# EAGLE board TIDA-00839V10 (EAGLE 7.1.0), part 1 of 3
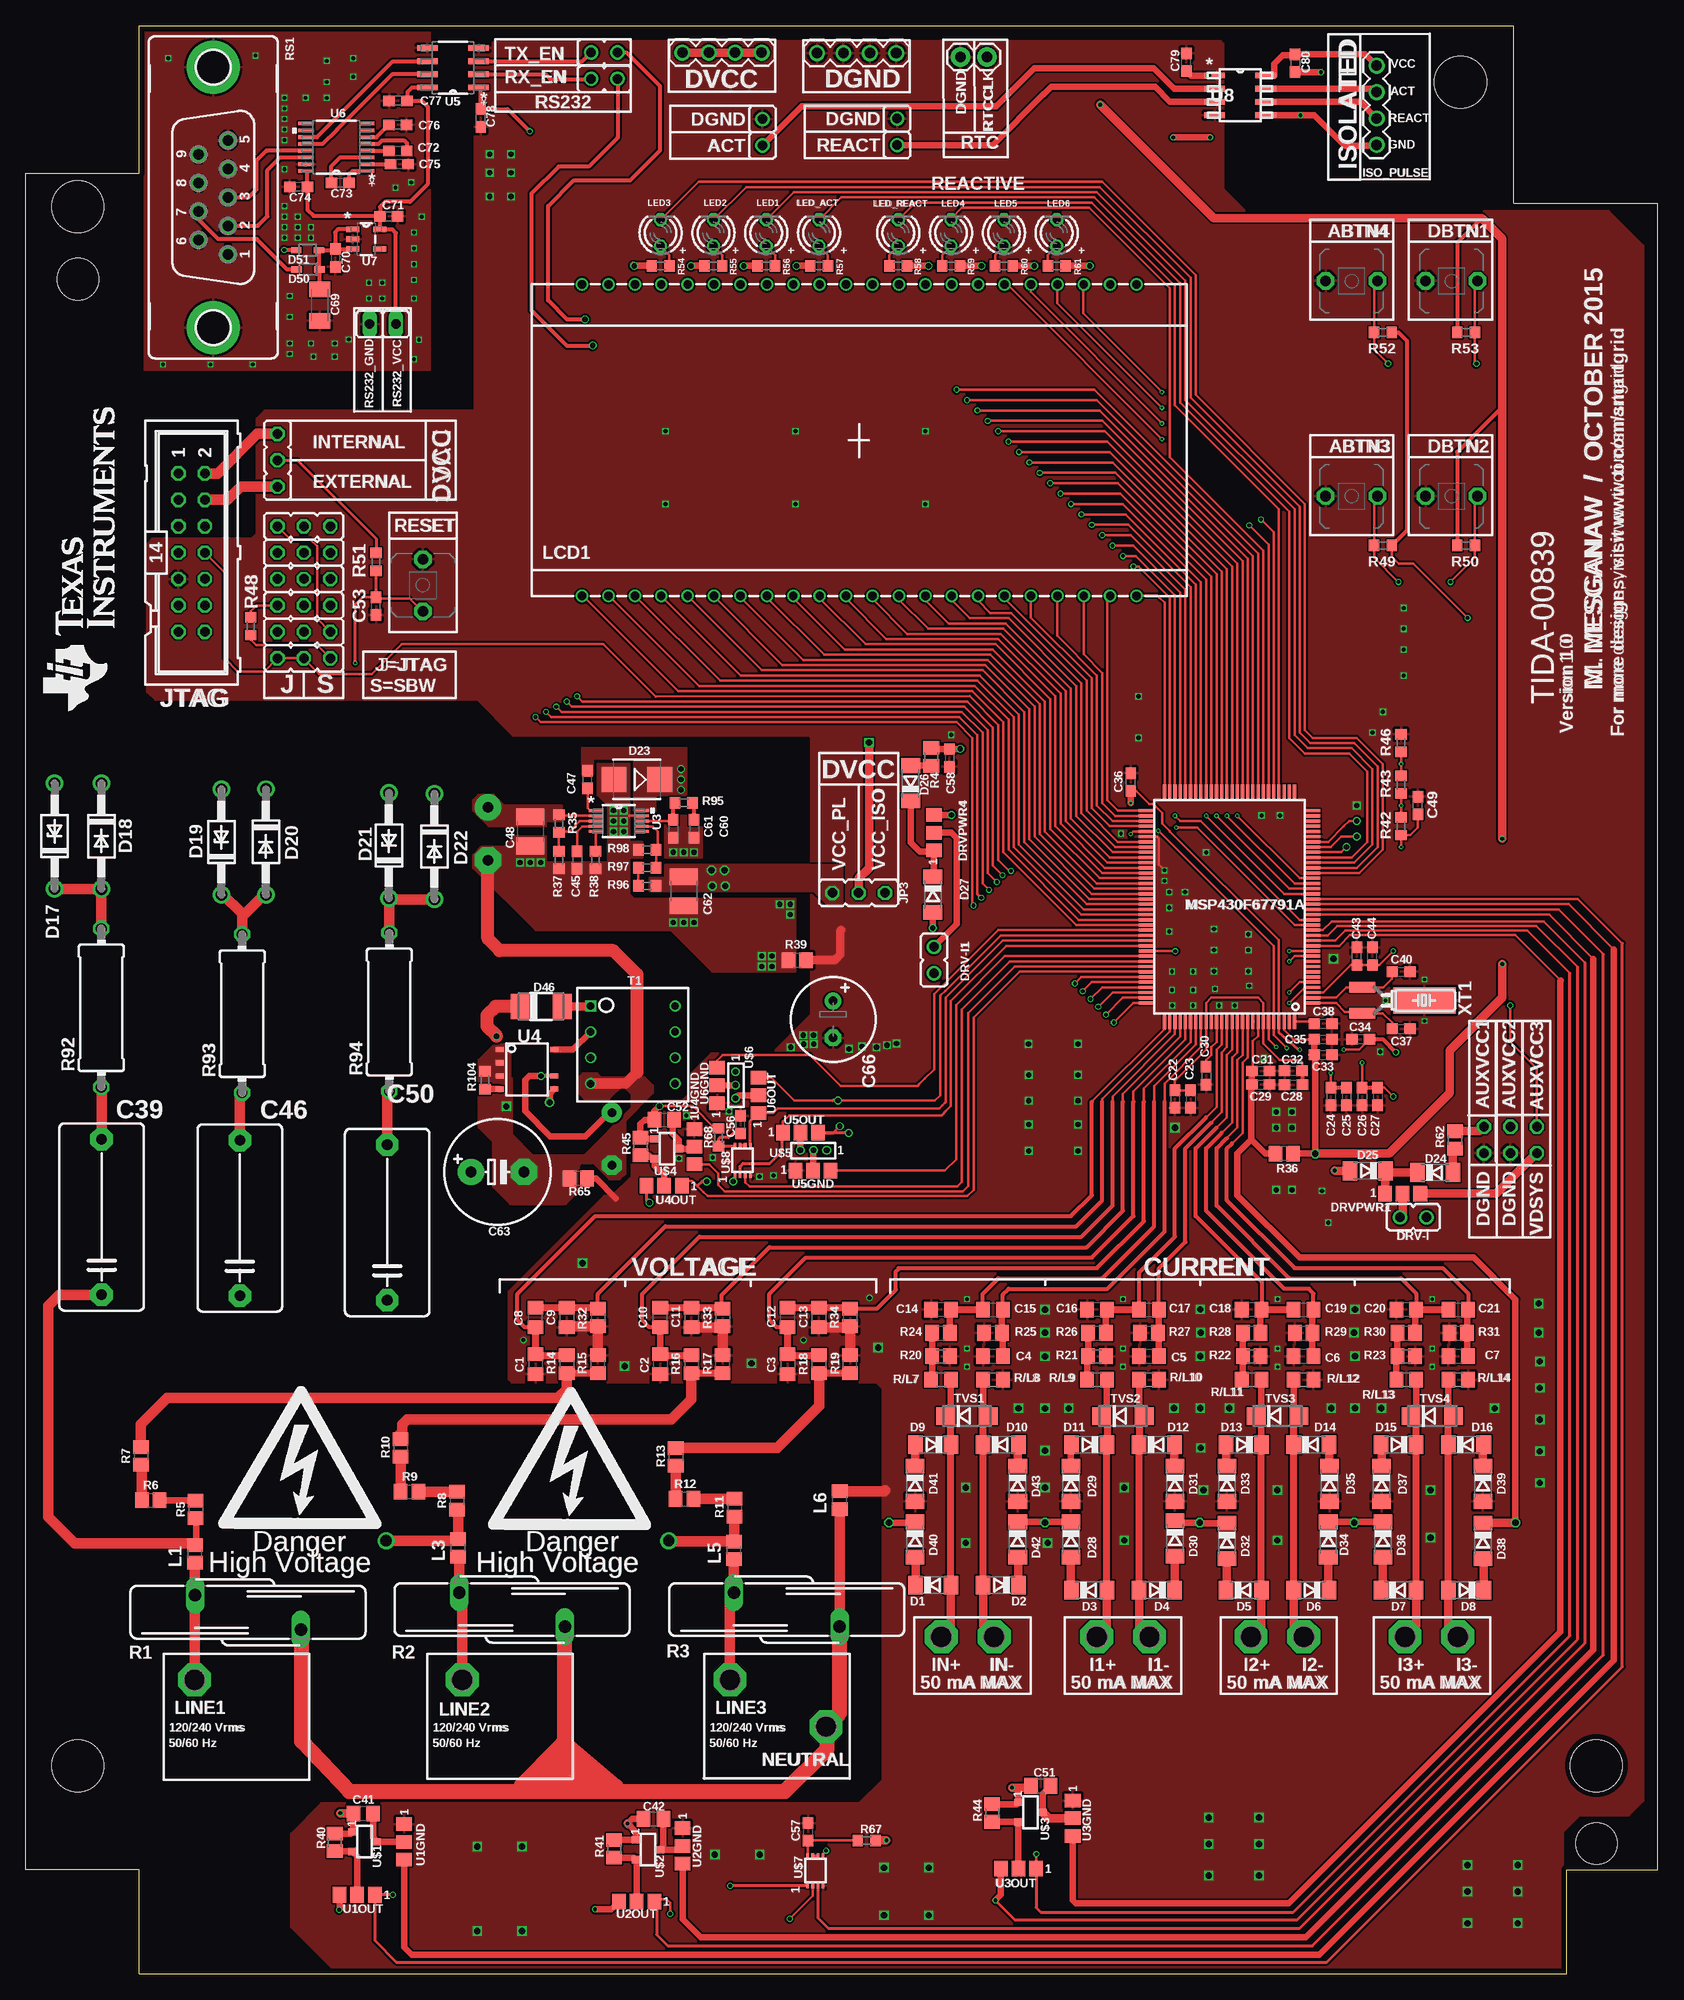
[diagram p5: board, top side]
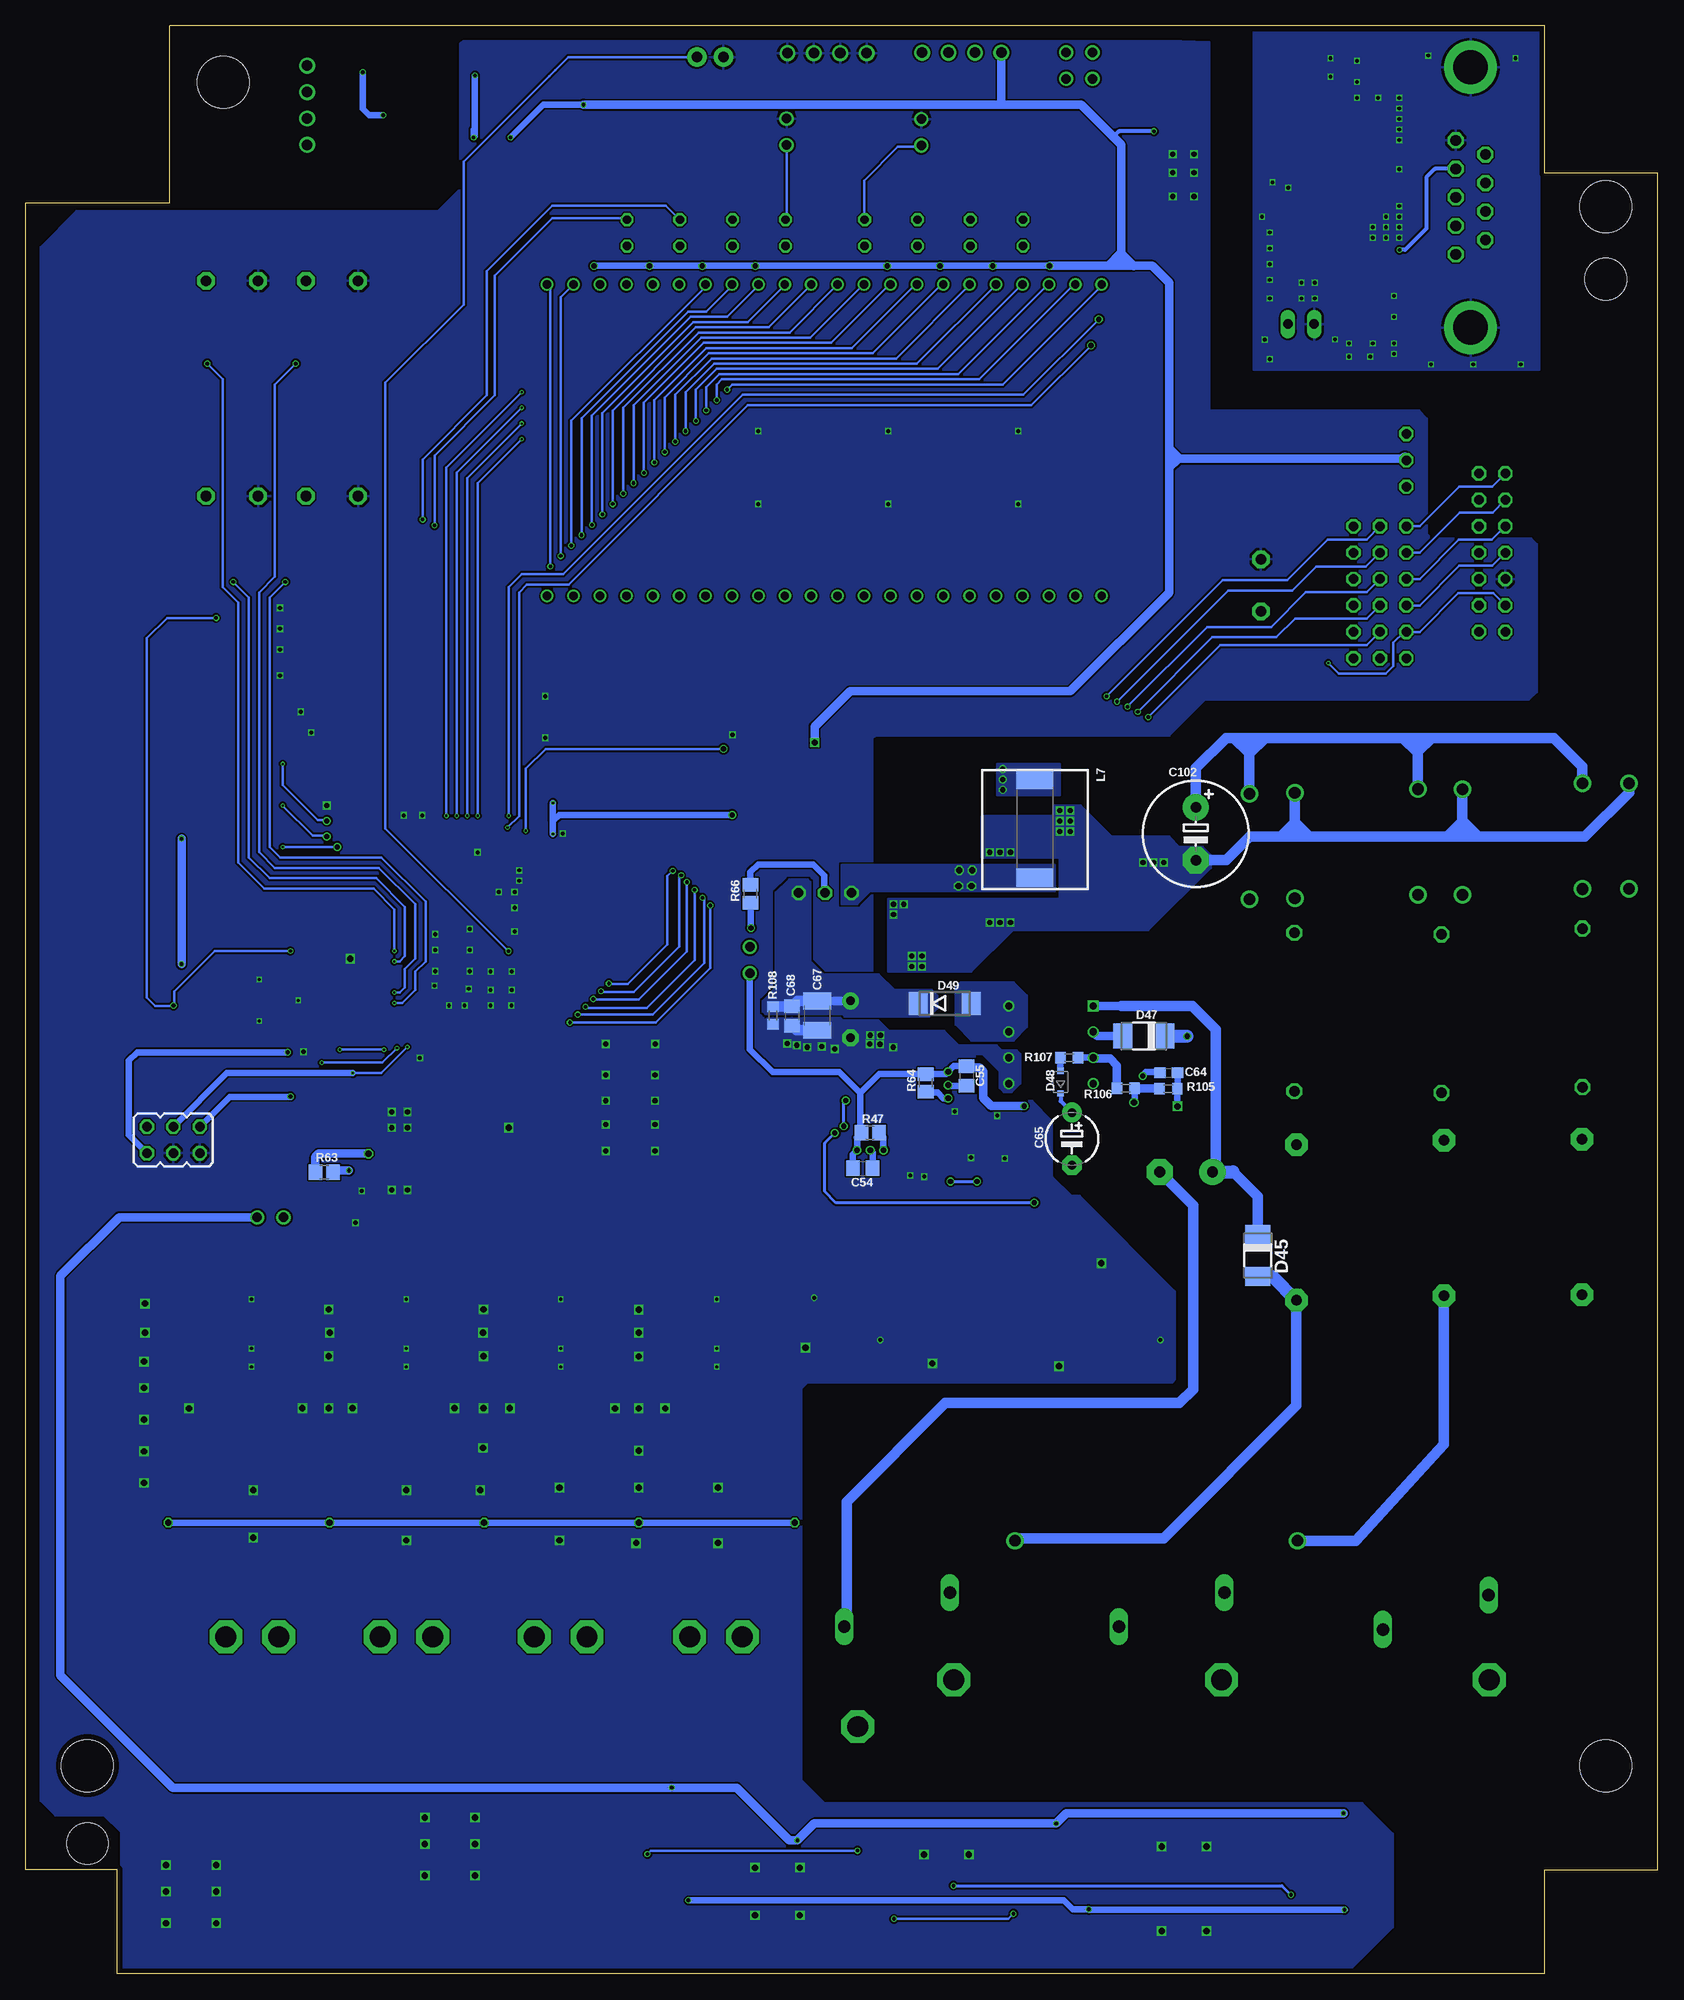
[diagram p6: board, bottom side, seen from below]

Size 156.94 x 187.36 mm. Coordinates in mm from the lower left corner, seen from the top.
Outline: 148.18,0 148.18,10 156.94,10 156.94,170.29 143.1,170.29 143.1,187.36 10.88,187.36 10.88,173.2 0,173.2 0,10 10.88,10 10.88,0 148.18,0
Copper layers (1*16): Top 0.0356mm / dielectric 1.5011mm / Bottom 0.0356mm
Design rules "SilverCircuits *": minimum track width 7mil, minimum drill 7.5mil, track to track 7mil, track to pad 7mil, pad to pad 7mil, via to via 7mil, smd to smd 0mil, copper to edge 20mil, drill to drill 8mil, minimum pad ring 5mil, minimum via ring 4mil, stop-mask expansion 4mil, vias tented up to drill 17mil, thermal gap 10mil
Holes 5 mm at 137.97,181.95 5,169.99 5,20 151.04,20
Holes 4 mm at 5,163 151.04,12.5

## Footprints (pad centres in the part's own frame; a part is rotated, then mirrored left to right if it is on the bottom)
PBTH = drill 1.016 pad 1.676 octagon: 1 -0.001,0.001; 2 5.001,0.001
C0805 = smd 1.3 x 1.5: 1 -0.95,0; 2 0.95,0
C0603 = smd 1.1 x 1: 1 -0.85,0; 2 0.85,0
C15B8 = drill 1.016 pad 2.159 octagon: 1 -7.493,0; 2 7.493,0
C1210 = smd 1.6 x 2.7: 1 -1.4,0; 2 1.4,0
E5-10,5 = drill 1.016 pad 2.54: + -2.54,0 | drill 1.016 pad 2.54 octagon: - 2.54,0
E5-5 = drill 0.813 pad 1.905: + -2.54,0 | drill 0.813 pad 1.905 octagon: - 2.54,0
E3,5-8 = drill 0.813 pad 1.6: + -1.778,0 | drill 0.813 pad 1.6 octagon: - 1.778,0
C1206K = smd 1.5 x 2: 1 -1.5,0; 2 1.5,0
SOD80C = smd 1.4 x 1.8: A 1.7,0; C -1.7,0
DO41Z10 = drill 1.118: A 5.08,0; C -5.08,0
DO41-10 = drill 1.118: A 5.08,0; C -5.08,0
SMB = smd 2.4 x 2.4: A 2.2,0; C -2.2,0
DO-214AC = smd 1.8 x 2.4: A 2.025,0; C -2.025,0
SOD323-R = smd 0.6 x 0.6: A 1.1,0; C -1.1,0
DO214AA = smd 1.8 x 2.2: A 2.55,0; C -2.55,0
SOD323 = smd 1 x 0.6: 1 -1.1,0; 2 1.1,0
MA04-1 = drill 1.016: 1 -3.81,0; 2 -1.27,0; 3 1.27,0; 4 3.81,0
JP1 = drill 0.914: 1 0,-1.27; 2 0,1.27
A0R-JMP = smd 1.5 x 1.3: 1 0,1.7; 2 0,0; 3 0,-1.7
P1-20 = drill 2.007 pad 3.15 octagon: TP 0,0
JP2 = drill 0.914 octagon: 1 -2.54,0; 2 0,0; 3 2.54,0
JP1' = drill 0.914 long: 1 0,-1.27; 2 0,1.27
ML14 = drill 0.914 octagon: 1 -7.62,-1.27; 2 -7.62,1.27; 3 -5.08,-1.27; 4 -5.08,1.27; 5 -2.54,-1.27; 6 -2.54,1.27; 7 0,-1.27; 8 0,1.27; 9 2.54,-1.27; 10 2.54,1.27; 11 5.08,-1.27; 12 5.08,1.27; 13 7.62,-1.27; 14 7.62,1.27
R0805 = smd 1.3 x 1.5: 1 -0.85,0; 2 0.85,0
INDUCTOR_POWER_SUPPLY_6779 = smd 3.556 x 1.778: 1 -3.81,-4.64; 2 -3.81,4.758
TI_160SEG_LCD = drill 0.8: 1 4.826,0; 2 7.366,0; 3 9.906,0; 4 12.446,0; 5 14.986,0; 6 17.526,0; 7 20.066,0; 8 22.606,0; 9 25.146,0; 10 27.686,0; 11 30.226,0; 12 32.766,0; 13 35.306,0; 14 37.846,0; 15 40.386,0; 16 42.926,0; 17 45.466,0; 18 48.006,0; 19 50.546,0; 20 53.086,0; 21 55.626,0; 22 58.166,0; 23 58.166,29.972; 24 55.626,29.972; 29 42.926,29.972; 30 40.386,29.972; 31 37.846,29.972; 32 35.306,29.972; 33 32.766,29.972; 34 30.226,29.972; 35 27.686,29.972; 36 25.146,29.972; 37 22.606,29.972; 38 20.066,29.972; 39 17.526,29.972; 40 14.986,29.972; 41 12.446,29.972; 42 9.906,29.972; 43 7.366,29.972; 44 4.826,29.972; COM0 45.466,29.972; COM1 48.006,29.972; COM2 50.546,29.972; COM3 53.086,29.972
LED3MM = drill 0.813 octagon: A -1.27,0; K 1.27,0
PEU128 = smd 0.3 x 1.4: 1 -9,-7.8; 2 -8.5,-7.8; 3 -8,-7.8; 4 -7.5,-7.8; 5 -7,-7.8; 6 -6.5,-7.8; 7 -6,-7.8; 8 -5.5,-7.8; 9 -5,-7.8; 10 -4.5,-7.8; 11 -4,-7.8; 12 -3.5,-7.8; 13 -3,-7.8; 14 -2.5,-7.8; 15 -2,-7.8; 16 -1.5,-7.8; 17 -1,-7.8; 18 -0.5,-7.8; 19 0,-7.8; 20 0.5,-7.8; 21 1,-7.8; 22 1.5,-7.8; 23 2,-7.8; 24 2.5,-7.8; 25 3,-7.8; 26 3.5,-7.8; 27 4,-7.8; 28 4.5,-7.8; 29 5,-7.8; 30 5.5,-7.8; 31 6,-7.8; 32 6.5,-7.8; 33 7,-7.8; 34 7.5,-7.8; 35 8,-7.8; 36 8.5,-7.8; 37 9,-7.8; 38 9.5,-7.8; 65 9.5,8.3; 66 9,8.3; 67 8.5,8.3; 68 8,8.3; 69 7.5,8.3; 70 7,8.3; 71 6.5,8.3; 72 6,8.3; 73 5.5,8.3; 74 5,8.3; 75 4.5,8.3; 76 4,8.3; 77 3.5,8.3; 78 3,8.3; 79 2.5,8.3; 80 2,8.3; 81 1.5,8.3; 82 1,8.3; 83 0.5,8.3; 84 0,8.3; 85 -0.5,8.3; 86 -1,8.3; 87 -1.5,8.3; 88 -2,8.3; 89 -2.5,8.3; 90 -3,8.3; 91 -3.5,8.3; 92 -4,8.3; 93 -4.5,8.3; 94 -5,8.3; 95 -5.5,8.3; 96 -6,8.3; 97 -6.5,8.3; 98 -7,8.3; 99 -7.5,8.3; 100 -8,8.3; 101 -8.5,8.3; 102 -9,8.3 | smd 1.4 x 0.3: 39 11.3,-6; 40 11.3,-5.5; 41 11.3,-5; 42 11.3,-4.5; 43 11.3,-4; 44 11.3,-3.5; 45 11.3,-3; 46 11.3,-2.5; 47 11.3,-2; 48 11.3,-1.5; 49 11.3,-1; 50 11.3,-0.5; 51 11.3,0; 52 11.3,0.5; 53 11.3,1; 54 11.3,1.5; 55 11.3,2; 56 11.3,2.5; 57 11.3,3; 58 11.3,3.5; 59 11.3,4; 60 11.3,4.5; 61 11.3,5; 62 11.3,5.5; 63 11.3,6; 64 11.3,6.5; 103 -10.8,6.5; 104 -10.8,6; 105 -10.8,5.5; 106 -10.8,5; 107 -10.8,4.5; 108 -10.8,4; 109 -10.8,3.5; 110 -10.8,3; 111 -10.8,2.5; 112 -10.8,2; 113 -10.8,1.5; 114 -10.8,1; 115 -10.8,0.5; 116 -10.8,0; 117 -10.8,-0.5; 118 -10.8,-1; 119 -10.8,-1.5; 120 -10.8,-2; 121 -10.8,-2.5; 122 -10.8,-3; 123 -10.8,-3.5; 124 -10.8,-4; 125 -10.8,-4.5; 126 -10.8,-5; 127 -10.8,-5.5; 128 -10.8,-6
S20K275 = drill 1.194 long: 1 -1.651,-5.08; 2 1.651,5.08
R0603 = smd 1 x 1.1: 1 -0.85,0; 2 0.85,0
0414/15 = drill 1.016 octagon: 1 -7.62,0; 2 7.62,0
R0805' = smd 1.3 x 1.5: 1 -0.95,0; 2 0.95,0
F09VP = drill 1.016 octagon: 1 5.486,1.422; 2 2.743,1.422; 3 0,1.422; 4 -2.743,1.422; 5 -5.486,1.422; 6 4.115,-1.422; 7 1.372,-1.422; 8 -1.372,-1.422; 9 -4.115,-1.422 | drill 3.302 pad 5.08: G1 -12.522,0; G2 12.522,0
1X02 = drill 1.016 pad 1.88: 1 0,0; 2 2.54,0
JP3Q = drill 0.914 octagon: 1 -2.54,-1.27; 2 -2.54,1.27; 3 0,-1.27; 4 0,1.27; 5 2.54,-1.27; 6 2.54,1.27
TRANS = drill 0.7 square: 1 -3.734,-4.064 | drill 0.7: 2 -1.245,-4.064; 3 1.245,-4.064; 4 3.734,-4.064; 5 3.734,4.064; 6 1.245,4.064; 7 -1.245,4.064; 8 -3.734,4.064
DO214AC = smd 1.8 x 1.7: A 2.05,0; C -2.05,0
DGQ10_1P88X1P57 = smd 1.422 x 0.279: 1 -2.184,0.991; 2 -2.184,0.508; 3 -2.184,0; 4 -2.184,-0.508; 5 -2.184,-0.991; 6 2.184,-0.991; 7 2.184,-0.508; 8 2.184,0; 9 2.184,0.508; 10 2.184,0.991
SOIC(D) = smd 0.5 x 0.75: 1 -1.905,-2.625; 2 -0.635,-2.625; 3 0.635,-2.625; 4 1.905,-2.625; 5 1.9,2.625; 6 0.635,2.625; 8 -1.905,2.625
SOIC127P600X175-8N = smd 1.981 x 0.559: 1 -2.464,1.905; 2 -2.464,0.635; 3 -2.464,-0.635; 4 -2.464,-1.905; 5 2.464,-1.905; 6 2.464,-0.635; 7 2.464,0.635; 8 2.464,1.905
SOP65P640X120-16N = smd 1.473 x 0.356: 1 -2.921,2.286; 2 -2.921,1.626; 3 -2.921,0.965; 4 -2.921,0.33; 5 -2.921,-0.33; 6 -2.921,-0.965; 7 -2.921,-1.626; 8 -2.921,-2.286; 9 2.921,-2.286; 10 2.921,-1.626; 11 2.921,-0.965; 12 2.921,-0.33; 13 2.921,0.33; 14 2.921,0.965; 15 2.921,1.626; 16 2.921,2.286
SOT95P280X145-5N = smd 1.27 x 0.559: 1 -1.295,0.94; 2 -1.295,0; 3 -1.295,-0.94; 4 1.295,-0.94; 5 1.295,0.94
D8 = smd 1.981 x 0.559: 1 -2.464,1.905; 2 -2.464,0.635; 3 -2.464,-0.635; 4 -2.464,-1.905; 5 2.464,-1.905; 6 2.464,-0.635; 7 2.464,0.635; 8 2.464,1.905
SOT23 = smd 0.7 x 0.8: 1 -0.92,-2.07; 2 0.98,-2.07; 3 0.03,0.275
SIP = drill 0.55: 1 0,0; 2 1.27,0; 3 2.54,0
DCU = smd 0.5 x 0.25: 1 1.39,-0.95; 2 1.39,-1.45; 3 1.39,-1.95; 4 1.39,-2.45; 5 4.29,-2.45; 6 4.29,-1.95; 7 4.29,-1.45; 8 4.29,-0.95
CM200T = smd 1 x 2.5: P1 -1.25,-5; P2 1.25,-5 | smd 2.5 x 6: P3 0,1

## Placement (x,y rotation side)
ABTN3  [PBTH]  125.01,142.13 0 top
ABTN4  [PBTH]  125.01,162.84 0 top
C1  47p  [C0805]  49.01,58.62 270 top
C2  47p  [C0805]  61.01,58.62 270 top
C3  47p  [C0805]  73.26,58.62 270 top
C4  47p  [C0805]  93.01,59.38 180 top
C5  47p  [C0805]  108.01,59.38 180 top
C6  47p  [C0805]  122.88,59.38 180 top
C7  47p  [C0805]  137.76,59.38 180 top
C8  15n  [C0805]  49.01,63.12 90 top
C9  47p  [C0805]  52.01,63.12 270 top
C10  15n  [C0805]  61.01,63.12 90 top
C11  47p  [C0805]  64.01,63.12 270 top
C12  15n  [C0805]  73.26,63.12 90 top
C13  47p  [C0805]  76.26,63.12 270 top
C14  47p  [C0805]  88.01,63.88 180 top
C15  15n  [C0805]  93.01,63.88 0 top
C16  47p  [C0805]  103.01,63.88 180 top
C17  15n  [C0805]  108.01,63.88 0 top
C18  47p  [C0805]  117.88,63.88 180 top
C19  15n  [C0805]  122.88,63.88 0 top
C20  47p  [C0805]  132.76,63.88 180 top
C21  15n  [C0805]  137.76,63.88 0 top
C22  4.7uF  [C0603]  110.51,84.12 270 top
C23  100nF  [C0603]  112.01,84.12 270 top
C24  4.7uF  [C0603]  125.51,84.38 270 top
C25  100nF  [C0603]  127.01,84.38 270 top
C26  4.7uF  [C0603]  128.51,84.38 270 top
C27  100nF  [C0603]  130.01,84.38 270 top
C28  100nF  [C0603]  121.91,85.5 180 top
C29  4.7uF  [C0603]  118.76,85.53 0 top
C30  100nF  [C0603]  113.51,86.38 270 top
C31  100nF  [C0603]  118.76,86.83 0 top
C32  4.7uF  [C0603]  121.9,86.83 180 top
C33  100nF  [C0603]  124.76,88.38 0 top
C34  4.7uF  [C0603]  128.38,89.88 180 top
C35  4.7uF  [C0603]  124.76,89.88 0 top
C36  100nF  [C0603]  106.26,114.62 90 top
C37  12pF  [C0603]  132.26,90.88 0 top
C38  0.47uF  [C0603]  124.76,91.38 0 top
C39  0.22uF/305VAC  [C15B8]  7.28,72.78 90 top
C40  12pF  [C0603]  132.26,96.38 0 top
C41  15n  [C0805]  32.43,15.4 0 top
C42  15n  [C0805]  60.35,14.89 0 top
C43  100nF  [C0603]  128.01,97.88 90 top
C44  0.47uF  [C0603]  129.51,97.88 90 top
C45  0.01uF  [C0603]  53.01,107.12 270 top
C46  0.22uF/305VAC  [C15B8]  20.57,72.69 90 top
C47  0.1uF  [C0603]  54.01,114.88 90 top
C48  2.2uF  [C1210]  48.51,109.88 270 top
C49  4.7uF  [C0603]  133.88,112.38 90 top
C50  0.22uF/305VAC  [C15B8]  34.75,72.25 90 top
C51  15n  [C0805]  97.59,18.06 0 top
C52  15n  [C0805]  61.4,82.14 0 top
C53  0.1uF  [C0603]  33.67,131.56 90 top
C54  15n  [C0805]  76.47,77.46 0 bottom
C55  15n  [C0805]  66.47,86.35 270 bottom
C56  4.7uF  [C0603]  68.73,81.67 90 top
C57  4.7uF  [C0603]  75.23,13.62 90 top
C58  DNP  [C0603]  88.82,116.95 270 top
C60  .056uF  [C0603]  64.26,110.12 270 top
C61  100pF  [C0603]  62.26,110.12 270 top
C62  47uF  [C1210]  63.26,104.12 270 top
C63  10u / 400V  [E5-10,5]  45.36,77.11 0 top
C64  0.1u  [C0603]  47.04,86.66 0 bottom
C65  18u  [E5-5]  56.34,80.29 270 bottom
C66  820u  [E3,5-8]  77.63,91.79 270 top
C67  10u  [C1210]  80.86,92.16 270 bottom
C68  0.1u  [C0805]  83.28,92.11 270 bottom
C69  47u  [C1206K]  28.26,160.5 270 top
C70  1u  [C0603]  29.77,165.04 270 top
C71  0.1u  [C0603]  34.89,169.05 0 top
C72  0.1u  [C0603]  35.77,175.35 0 top
C73  0.1u  [C0603]  30.22,172.26 180 top
C74  0.1u  [C0603]  26.22,171.88 180 top
C75  0.1u  [C0603]  35.91,174.07 180 top
C76  0.1u  [C0603]  35.75,177.85 180 top
C77  0.1u  [C0603]  35.78,180.16 180 top
C78  0.1u  [C0603]  43.74,178.52 90 top
C79  0.1u  [C0603]  111.61,183.87 90 top
C80  0.1u  [C0603]  122.07,183.78 270 top
C102  100uF/100V  [E5-10,5]  44.43,109.66 270 bottom
D1  PMLL4148  [SOD80C]  87.26,37.38 0 top
D2  PMLL4148  [SOD80C]  93.76,37.38 180 top
D3  PMLL4148  [SOD80C]  102.26,36.88 0 top
D4  PMLL4148  [SOD80C]  108.76,36.88 180 top
D5  PMLL4148  [SOD80C]  117.13,36.88 0 top
D6  PMLL4148  [SOD80C]  123.63,36.88 180 top
D7  PMLL4148  [SOD80C]  132.01,36.88 0 top
D8  PMLL4148  [SOD80C]  138.51,36.88 180 top
D9  PMLL4148  [SOD80C]  87.26,50.88 180 top
D10  PMLL4148  [SOD80C]  93.76,50.88 0 top
D11  PMLL4148  [SOD80C]  102.26,50.88 180 top
D12  PMLL4148  [SOD80C]  108.76,50.88 0 top
D13  PMLL4148  [SOD80C]  117.13,50.88 180 top
D14  PMLL4148  [SOD80C]  123.63,50.88 0 top
D15  PMLL4148  [SOD80C]  132.01,50.88 180 top
D16  PMLL4148  [SOD80C]  138.51,50.88 0 top
D17  1N4757A  [DO41Z10]  2.75,109.44 90 top
D18  1N4007  [DO41-10]  7.25,109.42 270 top
D19  1N4757A  [DO41Z10]  18.79,108.85 90 top
D20  1N4007  [DO41-10]  23.07,108.87 270 top
D21  1N4757A  [DO41Z10]  34.91,108.51 90 top
D22  1N4007  [DO41-10]  39.28,108.42 270 top
D23  B160  [SMB]  58.76,114.88 180 top
D24  PMLL4148  [SOD80C]  135.54,77.06 0 top
D25  PMLL4148  [SOD80C]  129.05,77.22 180 top
D26  PMLL4148  [SOD80C]  85.09,114.51 90 top
D27  PMLL4148  [SOD80C]  87.22,103.82 270 top
D28  PMLL4148  [SOD80C]  100.51,41.75 270 top
D29  PMLL4148  [SOD80C]  100.51,47.12 270 top
D30  PMLL4148  [SOD80C]  110.51,41.88 270 top
D31  PMLL4148  [SOD80C]  110.51,47.12 270 top
D32  PMLL4148  [SOD80C]  115.51,41.62 270 top
D33  PMLL4148  [SOD80C]  115.51,47.12 270 top
D34  PMLL4148  [SOD80C]  125.26,41.75 270 top
D35  PMLL4148  [SOD80C]  125.38,47.12 270 top
D36  PMLL4148  [SOD80C]  130.51,41.75 270 top
D37  PMLL4148  [SOD80C]  130.38,47.12 270 top
D38  PMLL4148  [SOD80C]  140.13,41.62 270 top
D39  PMLL4148  [SOD80C]  140.13,47.12 270 top
D40  PMLL4148  [SOD80C]  85.51,41.75 270 top
D41  PMLL4148  [SOD80C]  85.51,47.12 270 top
D42  PMLL4148  [SOD80C]  95.38,41.75 270 top
D43  PMLL4148  [SOD80C]  95.38,47.12 270 top
D45  US1J-E3/5AT  [DO-214AC]  38.46,69.08 270 bottom
D46  1SMB5954BT3G  [DO-214AC]  49.55,93.05 0 top
D47  US1M-13-F  [DO-214AC]  49.42,90.19 180 bottom
D48  BAS20HT1G  [SOD323-R]  57.44,85.76 90 bottom
D49  B130LB-13-F  [DO214AA]  68.58,93.33 0 bottom
D50  1N4148  [SOD323]  27.13,163.94 180 top
D51  1N4148  [SOD323]  27.09,165.8 180 top
DBTN1  [PBTH]  134.61,162.84 0 top
DBTN2  [PBTH]  134.61,142.13 0 top
DGND  [MA04-1]  79.9,184.75 0 top
DRV-I  [JP1]  133.44,72.74 90 top
DRV-I1  [JP1]  87.32,97.49 0 top
DRVPWR1  0R-JUMPA  [A0R-JMP]  132.4,75.03 270 top
DRVPWR4  0R-JUMPA  [A0R-JMP]  87.32,109.76 0 top
DVCC  [MA04-1]  66.94,184.8 0 top
I1+  TPPAD1-20  [P1-20]  102.99,32.39 90 top
I1-  TPPAD1-20  [P1-20]  108.07,32.39 90 top
I2+  TPPAD1-20  [P1-20]  117.81,32.39 90 top
I2-  TPPAD1-20  [P1-20]  122.89,32.39 90 top
I3+  TPPAD1-20  [P1-20]  132.64,32.39 90 top
I3-  TPPAD1-20  [P1-20]  137.72,32.39 90 top
IN+  TPPAD1-20  [P1-20]  88.04,32.39 90 top
IN-  TPPAD1-20  [P1-20]  93.12,32.39 90 top
ISO_PULSE  [MA04-1]  129.9,179.73 270 top
JP3  [JP2]  80.09,103.95 180 top
JP4  [JP2]  26.72,126.54 180 top
JP5  [JP2]  26.72,129.08 180 top
JP6  [JP2]  26.72,131.62 180 top
JP7  [JP2]  26.72,134.16 180 top
JP8  [JP2]  26.72,136.7 180 top
JP9  [JP2]  26.72,139.24 180 top
JP10  [JP2]  24.18,145.59 270 top
JP11  [JP1]  83.79,177.17 0 top
JP12  [JP1]  70.83,177.13 0 top
JP14  [JP1']  34.31,158.68 90 top
JTAG  [ML14]  15.93,136.7 270 top
L1  EXCML20A  [R0805]  16.24,40.38 90 top
L3  EXCML20A  [R0805]  41.57,40.96 90 top
L5  EXCML20A  [R0805]  68.11,40.71 90 top
L6  EXCML20A  [R0805]  78.27,45.53 90 top
L7  1mH  [INDUCTOR_POWER_SUPPLY_6779]  63.72,110.18 180 bottom
LCD1  TI_160SEG_LCD  [TI_160SEG_LCD]  48.65,132.53 0 top
LED1  [LED3MM]  71.2,167.46 90 top
LED2  [LED3MM]  66.12,167.46 90 top
LED3  [LED3MM]  61.04,167.46 90 top
LED4  [LED3MM]  88.98,167.46 90 top
LED5  [LED3MM]  94.06,167.46 90 top
LED6  [LED3MM]  99.14,167.46 90 top
LED_ACT  [LED3MM]  76.28,167.46 90 top
LED_REACT  [LED3MM]  83.9,167.46 90 top
LINE1  TPPAD1-20  [P1-20]  16.21,28.26 90 top
LINE2  TPPAD1-20  [P1-20]  41.96,28.26 90 top
LINE3  TPPAD1-20  [P1-20]  67.71,28.26 90 top
MSP430F67791A  MSP430F6779AIPEU  [PEU128]  116.01,102.38 90 top
NEUTRAL  TPPAD1-20  [P1-20]  76.95,23.76 90 top
R1  S20K275  [S20K275]  21.35,34.76 90 top
R2  S20K275  [S20K275]  46.75,35.01 90 top
R3  S20K275  [S20K275]  73.17,35.01 90 top
R4  0  [R0805]  87.07,117.05 90 top
R5  330k  [R0805]  16.32,44.65 270 top
R6  330k  [R0805]  12,45.54 0 top
R7  330k  [R0805]  11.05,49.79 270 top
R8  330k  [R0805]  41.45,45.49 270 top
R9  330k  [R0805]  36.89,46.36 0 top
R10  330k  [R0805]  36.02,50.57 270 top
R11  330k  [R0805]  68.13,44.82 270 top
R12  330k  [R0805]  63.34,45.66 0 top
R13  330k  [R0805]  62.49,49.7 270 top
R14  1k  [R0805]  52.01,58.62 270 top
R15  2.37K  [R0805]  55.01,58.62 90 top
R16  1k  [R0805]  64.01,58.62 270 top
R17  2.37K  [R0805]  67.01,58.62 90 top
R18  1k  [R0805]  76.26,58.62 270 top
R19  2.37K  [R0805]  79.26,58.62 90 top
R20  12.4  [R0805]  88.01,59.38 180 top
R21  12.4  [R0805]  103.01,59.38 180 top
R22  12.4  [R0805]  117.88,59.38 180 top
R23  12.4  [R0805]  132.76,59.38 180 top
R24  1k  [R0805]  88.01,61.62 0 top
R25  1k  [R0805]  93.01,61.62 0 top
R26  1k  [R0805]  103.01,61.62 0 top
R27  1k  [R0805]  108.01,61.62 0 top
R28  1k  [R0805]  117.88,61.62 0 top
R29  1k  [R0805]  122.88,61.62 0 top
R30  1k  [R0805]  132.76,61.62 0 top
R31  1k  [R0805]  137.76,61.62 0 top
R32  1k  [R0805]  55.01,63.12 270 top
R33  1k  [R0805]  67.01,63.12 270 top
R34  1k  [R0805]  79.26,63.12 270 top
R35  1M  [R0603]  51.26,110.62 90 top
R36  10R  [R0805]  121.02,78.89 180 top
R37  33.2K  [R0603]  51.26,107.12 90 top
R38  1M  [R0603]  54.76,107.12 90 top
R39  0  [R0805]  74.17,97.47 180 top
R40  30k  [R0805]  29.7,12.61 270 top
R41  30k  [R0805]  56.57,11.99 270 top
R42  560k  [R0603]  132.26,110.38 270 top
R43  560k  [R0603]  132.26,114.38 270 top
R44  30k  [R0805]  92.93,15.45 270 top
R45  30k  [R0805]  59.11,79.58 270 top
R46  560k  [R0603]  132.26,118.38 270 top
R47  30k  [R0805]  75.75,80.89 0 bottom
R48  330  [R0603]  21.62,129.62 270 top
R49  100K  [R0603]  130.51,137.38 180 top
R50  100K  [R0603]  138.51,137.38 0 top
R51  47K  [R0603]  33.67,135.81 270 top
R52  100K  [R0603]  130.51,157.88 180 top
R53  100K  [R0603]  138.51,157.88 0 top
R54  100  [R0603]  61.04,164.28 0 top
R55  100  [R0603]  66.12,164.28 0 top
R56  100  [R0603]  71.2,164.28 0 top
R57  100  [R0603]  76.28,164.28 0 top
R58  100  [R0603]  83.9,164.28 180 top
R59  100  [R0603]  88.98,164.28 180 top
R60  100  [R0603]  94.06,164.28 180 top
R61  100  [R0603]  99.14,164.28 180 top
R62  0  [R0805]  137.45,80.19 90 top
R63  0  [R0805]  128.26,77.1 180 bottom
R64  30k  [R0805]  70.4,85.69 270 bottom
R65  0  [R0805]  53.11,76.49 180 top
R66  0  [R0805]  87.27,103.87 90 bottom
R67  DNP  [R0603]  80.85,12.81 0 top
R68  DNP  [R0603]  66.62,80.45 90 top
R92  100  [0414/15]  7.24,92.9 90 top
R93  100  [0414/15]  20.8,92.34 90 top
R94  100  [0414/15]  34.95,92.5 90 top
R95  22.1k  [R0603]  63.26,112.62 180 top
R96  51.1  [R0603]  59.76,104.62 0 top
R97  31.6k  [R0603]  59.76,106.38 180 top
R98  10k  [R0603]  59.76,108.12 0 top
R104  2.87k  [R0603]  44.15,85.94 270 top
R105  30.1k  [R0603]  47.07,85.13 180 bottom
R106  76.8k  [R0603]  51.16,85.16 180 bottom
R107  10  [R0603]  56.6,88.1 0 bottom
R108  2.0k  [R0603]  85.1,92.17 90 bottom
R/L7  0  [R0805']  88.01,57.12 0 top
R/L8  0  [R0805']  93.01,57.12 180 top
R/L9  0  [R0805']  103.01,57.12 0 top
R/L10  0  [R0805']  108.01,57.12 180 top
R/L11  0  [R0805']  117.88,57.12 0 top
R/L12  0  [R0805']  122.88,57.12 180 top
R/L13  0  [R0805']  132.76,57.12 0 top
R/L14  0  [R0805']  137.76,57.12 180 top
RESET  [PBTH]  38.17,131.06 90 top
RS1  [F09VP]  18.01,170.88 270 top
RTC  [1X02]  89.88,184.36 0 top
RX_EN  [JP1]  55.63,182.28 270 top
SV1  [JP3Q]  142.77,80.2 0 bottom
T1  CUSTOMTRANS  [TRANS]  58.36,89.35 270 top
TVS1  SMAJ5.0CA  [DO214AC]  90.51,53.62 0 top
TVS2  SMAJ5.0CA  [DO214AC]  105.51,53.62 0 top
TVS3  SMAJ5.0CA  [DO214AC]  120.38,53.62 0 top
TVS4  SMAJ5.0CA  [DO214AC]  135.26,53.62 0 top
TX_EN  [JP1]  55.63,184.82 270 top
U1GND  0R-JUMPA  [A0R-JMP]  36.38,12.67 180 top
U1OUT  0R-JUMPA  [A0R-JMP]  31.86,7.58 90 top
U2GND  0R-JUMPA  [A0R-JMP]  63.15,12.29 180 top
U2OUT  0R-JUMPA  [A0R-JMP]  58.73,6.94 90 top
U3  TPS54060_DGQ_10  [DGQ10_1P88X1P57]  57.01,110.88 0 top
U3GND  0R-JUMPA  [A0R-JMP]  100.68,14.93 180 top
U3OUT  0R-JUMPA  [A0R-JMP]  95.46,10.09 90 top
U4  UCC28910D  [SOIC(D)]  48.19,86.98 270 top
U4GND  0R-JUMPA  [A0R-JMP]  64.29,79.54 180 top
U4OUT  0R-JUMPA  [A0R-JMP]  61.37,75.78 90 top
U5  ISO7421D  [SOIC127P600X175-8N]  41.08,183.35 180 top
U5GND  0R-JUMPA  [A0R-JMP]  75.7,77.25 270 top
U5OUT  0R-JUMPA  [A0R-JMP]  74.49,80.88 270 top
U6  TRS3232EQPWRQ1  [SOP65P640X120-16N]  29.85,175.69 180 top
U6GND  0R-JUMPA  [A0R-JMP]  66.47,85.45 0 top
U6OUT  0R-JUMPA  [A0R-JMP]  70.44,84.48 0 top
U7  TPS76333DBVT  [SOT95P280X145-5N]  32.72,166.85 0 top
U8  ISO7420_D_8  [D8]  116.78,180.69 0 top
U$1  DRV5033_SOT23  [SOT23]  33.47,12.71 270 top
U$2  DRV5033_SOT23  [SOT23]  60.72,11.94 270 top
U$3  DRV5033_SOT23  [SOT23]  97.52,15.54 270 top
U$4  DRV5033_SOT23  [SOT23]  62.53,79.38 270 top
U$5  DRV5033_SIP  [SIP]  77.01,79.22 180 top
U$6  DRV5033_SIP  [SIP]  68.25,86.74 270 top
U$7  SN74AUP2G32  [DCU]  74.22,7.04 90 top
U$8  SN74AUP2G32  [DCU]  67.23,75.38 90 top
XT1  [CM200T]  133.51,93.62 270 top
